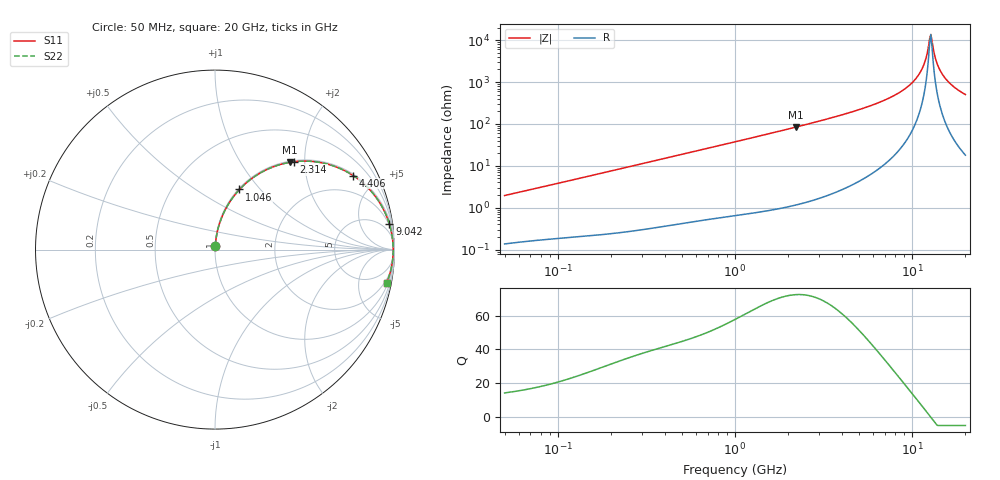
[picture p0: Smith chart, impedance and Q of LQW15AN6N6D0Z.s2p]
!Murata Part Number: LQW15AN6N6D0Z
!These Parameters are Measured in Series Mode Connection
!  o--[Z]--o
!Port1  Port2
!  o-------o
!Freq. Start=50[MHz] Stop=20[GHz], 401[Steps]
# Hz S RI R 50
!Freq.(Hz) S11(Real) S11(Imag) S21(Real) S21(Imag) S12(Real) S12(Imag) S22(Real) S22(Imag)
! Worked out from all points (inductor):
!   401 points, 50 MHz to 20 GHz, reference 50 ohm
!   read as one part in series: L = 6.15 nH near 51.52 MHz
!   highest Q = 72.5 at 2.212 GHz (marker M1), where L = 6.06 nH
!   self-resonance near 12.57 GHz
!   S11 on the Smith chart (normalised r, x): 50 MHz: 1.00, +0.04; 1.046 GHz: 1.01, +0.78; 2.314 GHz: 1.02, +1.77; 4.406 GHz: 1.06, +3.69; 9.042 GHz: 2, +13; 20 GHz: 1, -10
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5e7  0.00174 0.0194  0.9983 -0.0194  0.9983 -0.0194  0.00174 0.0194
1.364002e8  0.00471 0.0514  0.9953 -0.0514  0.9953 -0.0514  0.00471 0.0514
3.721004e8  0.0223 0.136  0.9777 -0.136  0.9777 -0.136  0.0223 0.136
1e9  0.1265 0.3238  0.8735 -0.3238  0.8735 -0.3238  0.1265 0.3238
1.045961e9  0.1364 0.3349  0.8636 -0.3349  0.8636 -0.3349  0.1364 0.3349
2.211938e9  0.4161 0.4861  0.5839 -0.4861  0.5839 -0.4861  0.4161 0.4861
2.313601e9  0.4392 0.4894  0.5608 -0.4894  0.5608 -0.4894  0.4392 0.4894
2.728004e9  0.5266 0.4923  0.4734 -0.4923  0.4734 -0.4923  0.5266 0.4923
4.405649e9  0.7692 0.4127  0.2308 -0.4127  0.2308 -0.4127  0.7692 0.4127
7.442007e9  0.939 0.2235  0.061 -0.2235  0.061 -0.2235  0.939 0.2235
9.041845e9  0.9713 0.1434  0.0287 -0.1434  0.0287 -0.1434  0.9713 0.1434
1.019291e10  0.9837 0.0934  0.0163 -0.0934  0.0163 -0.0934  0.9837 0.0934
1.115139e10  0.9895 0.0558  0.0105 -0.0558  0.0105 -0.0558  0.9895 0.0558
1.166392e10  0.9913 0.0369  0.00867 -0.0369  0.00867 -0.0369  0.9913 0.0369
1.201863e10  0.9921 0.0244  0.00787 -0.0244  0.00787 -0.0244  0.9921 0.0244
1.238412e10  0.9926 0.0118  0.00739 -0.0118  0.00739 -0.0118  0.9926 0.0118
1.276073e10  0.9928 -0.000774  0.00724 0.000774  0.00724 0.000774  0.9928 -0.000774
1.295331e10  0.9927 -0.00706  0.00728 0.00706  0.00728 0.00706  0.9927 -0.00706
1.396067e10  0.9913 -0.0385  0.00868 0.0385  0.00868 0.0385  0.9913 -0.0385
1.482269e10  0.9887 -0.0636  0.0113 0.0636  0.0113 0.0636  0.9887 -0.0636
1.696185e10  0.9782 -0.1201  0.0218 0.1201  0.0218 0.1201  0.9782 -0.1201
2e10  0.9557 -0.1886  0.0443 0.1886  0.0443 0.1886  0.9557 -0.1886
